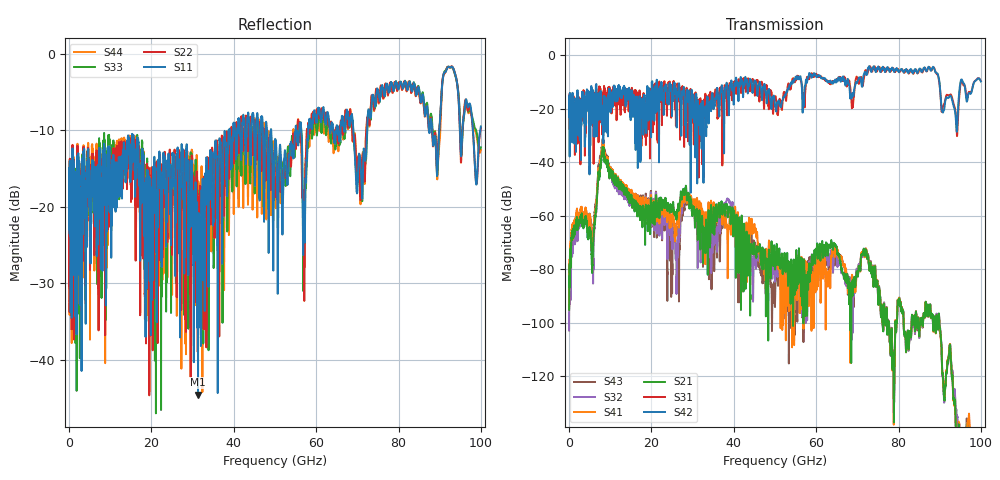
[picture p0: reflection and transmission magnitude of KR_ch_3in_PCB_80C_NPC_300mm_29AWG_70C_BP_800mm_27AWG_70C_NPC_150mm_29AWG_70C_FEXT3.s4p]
# Hz S RI R 45
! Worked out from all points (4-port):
!   4000 points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, 25 MHz to 100 GHz, reference 45 ohm
!   strongest paths, dB at 25 MHz, 25.02 GHz, 50.02 GHz, 75.03 GHz, 100 GHz:
!     S42: -20.7, -20.7, -18.8, -4.2, -9.7
!     S31: -20.7, -14.8, -15.8, -5.0, -9.6
!     S21: -95.2, -57.5, -78.7, -90.8, -159.1
!     S41: -94.5, -61.5, -78.3, -90.7, -154.9
!     S32: -103.0, -67.2, -81.9, -90.6, -161.2
!     S43: -95.1, -89.0, -92.1, -90.5, -165.4
!   lowest |S11| = -44.5 dB at 31.32 GHz (marker M1), VSWR 1.01, Z = 44.5 - j0.116 ohm
!   |S11| at or under -10 dB: start of sweep to 38.74 GHz; 49.09 GHz to 54.99 GHz (5.9 GHz wide, 11.3 % of centre); 69.01 GHz to 72.38 GHz (3.369 GHz wide, 4.77 % of centre)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
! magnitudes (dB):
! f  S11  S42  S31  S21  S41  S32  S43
! 25 MHz  -16.6  -20.7  -20.7  -95.2  -94.5  -103.0  -95.1
! 5.825 GHz  -15.1  -14.9  -16.7  -71.6  -68.4  -83.9  -67.3
! 8.225 GHz  -16.1  -21.2  -15.1  -34.5  -32.9  -33.0  -31.6
! 24.68 GHz  -19.0  -12.6  -14.3  -56.0  -60.6  -65.1  -71.3
! 31.32 GHz  -44.5  -18.5  -21.1  -60.4  -55.6  -62.5  -57.1
! 46.83 GHz  -8.3  -16.1  -10.0  -79.9  -76.9  -77.5  -80.3
! 100 GHz  -9.5  -9.7  -9.6  -159.1  -154.9  -161.2  -165.4
